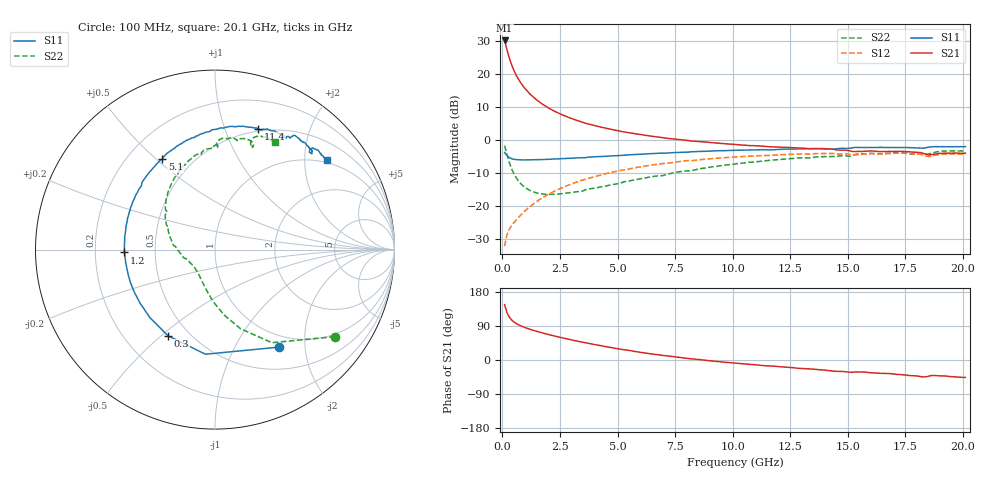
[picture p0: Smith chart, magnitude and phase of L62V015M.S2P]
!  Infineon Technologies AG
! BFR380L3 , PF131585-7, No.6, Th 09.10.01, soldered on pcb-board, measured with PP GSG850
!  Vce=2.0 V,  Ic=15.0 mA
! Common Emitter S-Parameters:  15. November 2001
#  GHz  S  MA  R  50
! f  S11  S21  S12  S22
! GHz  Mag  Ang  Mag  Ang  Mag  Ang  Mag  Ang
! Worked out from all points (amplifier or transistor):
!   201 points, 100 MHz to 20.1 GHz, reference 50 ohm
!   highest |S21| = 30.1 dB at 100 MHz (marker M1)
!   |S21| within 3 dB of that: start of sweep to 210.3 MHz
!   unconditionally stable (mu >= 1): 1.546 GHz to 4.573 GHz
!   at 3.4 GHz: K = 1.02, MAG = 8.0 dB, |S12| = -12.3 dB
!   at 10.1 GHz: K = 0.96, MSG = 1.9 dB, |S12| = -5.1 dB
!   at 20.1 GHz: K = 0.99, MSG = 0.1 dB, |S12| = -4.1 dB
!   S11 on the Smith chart (normalised r, x): 100 MHz: 0.82, -1.53; 300 MHz: 0.38, -0.53; 1.2 GHz: 0.33, -0.01; 5.1 GHz: 0.34, +0.52; 11.4 GHz: 0.47, +1.31; 20.1 GHz: 0.92, +2.55
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0.1  0.6502 -56.6  32 146.1  0.02502 64.5  0.825 -36.0
0.2  0.5854 -95.2  23.33 125.3  0.03709 55.2  0.608 -58.6
0.3  0.5467 -118.7  17.54 113.6  0.04485 51.5  0.4632 -72.1
0.4  0.5248 -133.5  13.85 106.0  0.05069 51.4  0.3718 -81.5
0.5  0.5132 -144.4  11.37 100.6  0.05636 52.8  0.3121 -88.7
0.6  0.5083 -152.2  9.614 96.5  0.06221 54.1  0.2715 -94.6
0.7  0.5058 -158.4  8.331 93.1  0.06799 55.5  0.2416 -99.7
0.8  0.5036 -163.6  7.34 90.1  0.07391 56.9  0.22 -104.2
0.9  0.5017 -168.0  6.56 87.6  0.07997 57.8  0.2034 -108.2
1  0.5027 -171.7  5.937 85.2  0.08621 58.7  0.1912 -112.0
1.2  0.5045 -178.2  4.985 81.0  0.09892 59.9  0.1739 -118.7
1.6  0.5079 171.9  3.788 73.7  0.1253 60.9  0.1569 -129.8
2.1  0.5144 161.9  2.934 65.8  0.1585 60.1  0.152 -140.9
2.7  0.526 151.5  2.332 57.2  0.198 57.9  0.157 -152.2
3.5  0.5416 139.8  1.852 46.7  0.2505 53.8  0.1707 -163.3
5.1  0.5843 120.1  1.368 28.7  0.3481 43.5  0.2222 175.3
6.8  0.6323 102.5  1.106 13.2  0.4357 32.3  0.2896 154.6
10.1  0.7011 78.2  0.8582 -8.2  0.5559 10.9  0.4369 124.1
11.4  0.7147 70.4  0.8047 -15.1  0.5855 2.6  0.4874 113.1
13.5  0.7395 60.5  0.748 -24.4  0.6208 -9.6  0.5494 97.4
16.8  0.7756 48.2  0.678 -35.8  0.6264 -25.4  0.6351 76.8
20.1  0.7983 38.8  0.635 -46.1  0.6202 -39.0  0.6896 60.8
